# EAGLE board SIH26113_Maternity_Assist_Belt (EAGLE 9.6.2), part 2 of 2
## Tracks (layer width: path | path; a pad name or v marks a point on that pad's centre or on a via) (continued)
LED_STDBY_K  (via drill 0.3 pad 0.6)
  Top 0.2: 24.8,14.6 24.8,15 25,15.2 25,20 24.8,20.2 24.2,20.8 24,21 24,21.4 23.6,21.4 23.2,21.8 23,22 22.8,22.2 v22.4,22.6
  Top 0.25: U1.6 24.6,14.37
  Bottom 0.2: v22.4,22.6 22.2,22.8 22,23 21.8,23.2 21.2,23.8 21,24 20.8,24.2 v20.2,24.8
MOTOR_EN  (via drill 0.3 pad 0.6)
  Top 0.2: 69.6,59.6 69.6,59.8 69.8,60 70.2,60.4 70.4,60.6 70.6,60.8 70.8,61 71.2,61.4 71.2,64.4 71,64.6 70.8,64.8 | 23,45.6 23,47.4 22.8,47.6 22.6,47.8 22.4,48 v22.2,48.2 | v21.6,48.8 21.6,49 22,49.4 22.2,49.6 22.4,49.8 v22.4,55 | v22.4,55.8 22.6,56 23,56.4 23.2,56.6 23.4,56.8 23.6,57 24,57.4 24.2,57.6 24.4,57.8 24.6,58 v25,58.4 | v31,61.4 36.2,61.4 36.6,61.8 36.8,62 37.8,62 38,62.2 38.2,62.4 38.4,62.6 38.6,62.8 38.8,63 v41.2,63 | v56,62.6 67,62.6 67.2,62.8 67.4,63 67.6,63.2 67.8,63.4 68,63.6 68.2,63.8 68.4,64 68.6,64.2 68.8,64.4 69,64.6 69.2,64.8
  Top 0.25: U3.24 23.45,41.15
  Bottom 0.2: v22.2,48.2 22,48.4 21.8,48.6 v21.6,48.8 | v22.4,55 v22.4,55.8 | v25,58.4 25.2,58.6 25.4,58.8 25.6,59 26,59.4 26,60.4 29.8,60.4 30,60.6 30.2,60.8 30.4,61 30.8,61.4 v31,61.4 | v41.2,63 41.4,62.8 41.6,62.8 41.8,62.6 v56,62.6
MOTOR_G
  Top 0.2: 71.6,58.2 71.6,57.6 71.8,57.4 72,57.2 | 72,57.2 72,55.8 71.6,55.8 71.4,55.6 71.2,55.4 71,55.4 70.8,55.2 | 73.8,57.4 72.2,57.4 72,57.2
MOTOR_N
  Top 0.5: 83,62.8 83,64.8 84.4,66.2 | 75.2,60.6 81,60.6 81.2,60.8 81.4,61 81.8,61.4 82,61.6
MOTOR_P  (via drill 0.3 pad 0.6)
  Top 0.5: 80,64.8 80.4,64.8 80.8,65.2 81,65.4 81.2,65.6 81.4,65.8 81.8,66.2 82,66.4 82.2,66.6 82.4,66.8 82.8,67.2 83,67.4 83.2,67.6 83.4,67.8 83.8,68.2 84,68.4 85.6,68.4 85.8,68.2 86,68 86.2,67.8 86.4,67.6 86.4,67.4 | 75.6,62.4 75.6,62.2 77.8,62.2 78,62.4 78.2,62.6 78.6,62.6 78.8,62.8 78.8,63.2
  Bottom 0.5: v82,60.4 82,61.2 81.8,61.4 81.6,61.6 81.4,61.8 81.2,62 81,62.2 80.8,62.4 80.6,62.6 80.4,62.8 80.2,63 v80,63.2
PIEZO_AC  (via drill 0.3 pad 0.6)
  Top 0.2: 56.8,6.8 56.8,7.2 56.6,7.4 56.4,7.6 56.2,7.8 v56,8 | 57.2,17 v57.2,16.4 | 55,18.8 55.2,18.6 55.4,18.6 55.6,18.4 55.8,18.2 56,18.2
  Bottom 0.2: v56,8 55.8,8.2 55.8,10.4 v55.6,10.6 | v57.2,16.4 57.2,13.2 57,13 56.8,12.8 56.6,12.6 56.4,12.4 56.2,12.2 56,12 v55.6,12
PIEZO_ADC  (via drill 0.3 pad 0.6)
  Top 0.2: 58.8,14.4 v58.8,12.6 | 59.6,21.2 v60.2,21.2 | 54.6,21.8 v54.8,21.8 | 33.2,59.8 33.4,59.6 33.6,59.4 33.8,59.2 34,59 34.2,58.8 34.4,58.6 34.6,58.4 v34.8,58.2 | v48.2,61 53.6,61 53.8,60.8 v57.4,60.8 | v63.6,60.8 63.8,60.6 65.4,60.6 65.6,60.4 v65.6,55.8 | v65.6,25 65.2,25 65,25.2 64.8,25.4 63.6,25.4 63.4,25.2 63.2,25 63,24.8 62.8,24.6 62.6,24.4 62.4,24.2 62.2,24 62,23.8 61.8,23.6 61.6,23.4 61.4,23.2 61.2,23 61,22.8 60.8,22.6 60.6,22.4 59.6,22.4
  Top 0.25: U3.38 33.05,59.97
  Bottom 0.2: v58.8,12.6 58.8,12.2 58.6,12 v58.6,6.8 | v60.2,21.2 60.6,21.2 60.8,21 60.8,18.4 60.6,18.2 60.4,18 60,17.6 v60,15.6 | v54.8,21.8 v58.4,21.8 | v34.8,58.2 35,58 35.2,57.8 38.8,57.8 42.4,61.4 42.8,61.4 43.2,61.8 46.4,61.8 46.6,61.6 46.8,61.4 47,61.2 47.2,61 v48.2,61 | v57.4,60.8 v63.6,60.8 | v65.6,55.8 65.6,52.6 65.4,52.4 65,52 65,50.4 65.4,50 65.6,49.8 65.8,49.6 65.8,49 66,48.8 66.2,48.6 66.2,40.6 66,40.4 65.8,40.2 65.8,30 66.2,29.6 66.2,27.8 66,27.6 66,25.2 65.8,25 v65.6,25
PIEZO_IN  (via drill 0.3 pad 0.6)
  Top 0.2: 54.4,6.4 54.4,3.8 | 53.6,10.6 53.8,10.4 54,10.2 v54.2,10
  Bottom 0.2: v54.2,10 54.4,9.8 54.6,9.6 v54.6,7.6
SD_CS
  Top 0.25: U3.18 15.82,41.15
SD_MISO
  Top 0.25: U3.21 19.64,41.15
SD_MOSI  (via drill 0.3 pad 0.6)
  Top 0.2: 17.2,39.2 19.6,39.2 19.8,39 20,38.8 20.2,38.6 20.4,38.4 22.8,38.4 23,38.2 23.2,38 23.4,37.8 23.8,37.4 24,37.2 24.2,37 24.4,36.8 24.8,36.4 25,36.2 25.2,36 25.4,35.8 25.8,35.4 26,35.2 26.2,35 26.4,34.8 26.8,34.4 27,34.2 27.2,34 27.4,33.8 27.8,33.4 28,33.2 28.2,33 28.4,32.8 28.8,32.4 29,32.2 30.8,30.4 31,30.4 31.2,30.2 31.4,30 32,29.4 32.2,29.2 32.4,29 32.8,28.6 33,28.4 33.2,28.2 33.4,28 33.6,27.8 33.6,27.4 33.8,27.2 34,27 34,26.4 34.2,26.2 34.4,26 34.8,25.6 36.8,25.6 37,25.4 37.2,25.2 37.4,25 37.8,24.6 38,24.4 38.2,24.2 38.4,24 38.6,23.8 38.8,23.6 39,23.4 v39.2,23.2 | v42,22.4 42,24 42.2,24.2 42.4,24.4 42.6,24.6 42.8,24.8 v43,25 | v43.6,25.6 v45,25.6 | v52.4,23.2 55,23.2 55,25 55.2,25.2 55.4,25.4 55.6,25.6 55.8,25.8 56,26 56.2,26.2 56.4,26.4 56.6,26.6 56.8,26.8 57,27 57.2,27.2 57.4,27.4 57.6,27.6 57.8,27.8 58,28 58.2,28.2 58.4,28.4 58.6,28.6 58.8,28.8 59,29 59.2,29.2 59.4,29.4 59.6,29.6 59.8,29.8 60,30 60.2,30.2 60.4,30.4 60.6,30.6 v60.8,30.8 | v62.8,32 63,32.2 63.2,32.4 63.4,32.6 63.6,32.8 63.8,33 64,33.2 64.2,33.4 64.6,33.8 v64.6,48 | v64,59 63,59 62.8,59.2 62.4,59.6 62.2,59.6 61.6,60.2 61.4,60.4 61.2,60.6 60.6,61.2 60.4,61.4 60.2,61.6 59.8,62 53.4,62 51,64.4 50.8,64.6 50.6,64.8 50.4,64.8 50.2,65 49.6,65 49.4,65.2 v49.2,65.4
  Top 0.25: U3.19 17.09,39.45
  Bottom 0.2: v39.2,23.2 39.4,23 39.6,22.8 39.8,22.6 40,22.4 40.2,22.2 40.4,22 40.6,21.8 40.8,21.6 42,21.6 v42,22.4 | v43,25 43.2,25.2 43.4,25.4 v43.6,25.6 | v45,25.6 50,25.6 50.4,25.2 50.6,25 50.8,24.8 51,24.6 51.4,24.2 51.6,24 51.8,23.8 52,23.6 v52.4,23.2 | v60.8,30.8 61,31 61.2,31.2 61.4,31.4 61.6,31.6 61.8,31.8 62,32 v62.8,32 | v64.6,48 64.6,49.6 64.4,49.8 64.4,58.6 64.2,58.8 v64,59 | v49.2,65.4 49,65.6 48.8,65.8 48.6,66 48.4,66.2 48,66.6
SD_SCK  (via drill 0.3 pad 0.6)
  Top 0.2: v17.8,46.8 18.6,46.8 18.8,47 20.4,47 20.8,47.4 21,47.6 21.2,47.8 21.4,48 21.8,48.4 22,48.6 22.2,48.8 22.4,49 22.8,49.4 23,49.6 23.2,49.8 23.4,50 23.8,50.4 24,50.6 24.2,50.8 24.4,51 24.8,51.4 v25,51.6
  Top 0.25: U3.20 18.36,42.85
  Bottom 0.2: v18,45.6 18,46.4 17.8,46.6 v17.8,46.8 | v25,51.6 25.2,51.8 25.4,52 25.8,52.4 26,52.6 27.4,52.6 27.6,52.8 27.8,53 28,53.2 28.2,53.4 28.4,53.6 28.6,53.8 28.8,54 29,54.2 29.2,54.4 29.4,54.6 29.6,54.8 29.8,55 30,55.2 30.2,55.4 30.4,55.6 30.6,55.8 30.8,56 31,56.2 31.2,56.4 31.4,56.6 31.6,56.8 31.8,57 32,57.2 32.6,57.8 32.8,58 33,58.2 33.6,58.8 33.8,59 34,59.2 34.6,59.8 34.8,60 35,60.2 35.2,60.2 35.4,60.4 37,60.4 37.2,60.6 37.4,60.8 37.6,61 37.8,61.2 38,61.4 38.2,61.6 38.8,62.2 39,62.4 39.2,62.6 39.8,63.2 40,63.4 40.2,63.6 40.8,64.2 41,64.4 41.2,64.6 41.4,64.8 41.6,64.8 41.8,65 42.4,65 42.6,65.2 42.8,65.4 43,65.6 43.2,65.8 43.4,66 43.6,66.2 43.8,66.4 44,66.6
SOS_BTN
  Top 0.2: 49.6,57.4 49.6,58.2 49.8,58.4 | 52.8,55.2 49.8,55.2 49.8,55.8 49.6,56 | 58,61.6 52.8,61.6 50.6,63.8
SOS_GPIO  (via drill 0.3 pad 0.6)
  Top 0.2: 51.6,57.4 51.6,57.6 v53.4,59.4 | 29.8,53.8 v33,53.8
  Top 0.25: U3.33 29.65,53.62
  Bottom 0.2: v53.4,59.4 56.8,62.8 57,62.8 57.2,63 57.2,63.2 57.4,63.4 57.4,63.6 57.6,63.8 57.8,64 v58,64.2 | v33,53.8 48.2,53.8 48.4,54 48.6,54.2 49.2,54.8 49.4,55 49.6,55.2 50.2,55.8 v50.4,56
STRETCH_ADC  (via drill 0.3 pad 0.6)
  Top 0.2: 58.8,10.2 59.6,10.2 59.8,10.4 60,10.6 60.2,10.8 | 56.8,13 56.8,10.4 57,10.4 57.2,10.2 | v31.6,31.2 31.8,31 32,30.8 32.2,30.6 32.4,30.4 32.6,30.2 32.8,30 33,29.8 33.2,29.6 33.4,29.4 33.6,29.2 33.8,29 34,28.8 34.2,28.6 34.4,28.4 34.6,28.2 34.8,28 37,28 37.2,27.8 37.4,27.6 37.8,27.2 38,27 38.4,26.6 38.6,26.4 38.8,26.2 39,26 39.4,25.6 39.6,25.4 39.8,25.2 40,25 v40.2,24.8 | v43.6,21.4 43.8,21.2 44,21 v44.2,20.8
  Top 0.25: U3.12 4.95,48.54
  Bottom 0.2: v11,48 14.8,48 15,47.8 15.2,47.6 15.4,47.4 15.6,47.2 15.8,47 16,46.8 16.2,46.6 16.4,46.4 16.8,46 17,45.8 17.2,45.6 17.4,45.4 17.8,45 18,44.8 18.2,44.6 18.4,44.4 18.8,44 19,43.8 19.2,43.6 19.4,43.4 19.8,43 20,42.8 20.2,42.6 20.4,42.4 20.8,42 21,41.8 21.2,41.6 21.4,41.4 21.8,41 22,40.8 22.2,40.6 22.4,40.4 22.8,40 23,39.8 23.2,39.6 23.4,39.4 23.8,39 24,38.8 24.2,38.6 24.4,38.4 24.8,38 25,37.8 25.2,37.6 25.4,37.4 25.6,37.2 25.8,37 26,36.8 26.2,36.6 26.4,36.4 26.6,36.2 26.8,36 27,35.8 27.2,35.6 27.4,35.4 27.6,35.2 27.8,35 28,34.8 28.2,34.6 28.4,34.4 28.6,34.2 28.8,34 29,33.8 29.2,33.6 29.4,33.4 29.6,33.2 29.8,33 30,32.8 30.2,32.6 30.4,32.4 30.6,32.2 30.8,32 31,31.8 31.2,31.6 v31.6,31.2 | v40.2,24.8 40.4,24.6 40.6,24.4 40.8,24.2 41,24 41.4,23.6 41.6,23.4 41.8,23.2 42,23 42.4,22.6 42.6,22.4 42.8,22.2 43,22 43.4,21.6 v43.6,21.4 | v44.2,20.8 46.4,20.8 46.6,20.6 46.8,20.4 47,20.2 47.2,20 47.4,19.8 47.6,19.6 47.8,19.4 48,19.2 48.2,19 48.4,18.8 48.6,18.6 48.8,18.4 49,18.2 49.4,17.8 49.6,17.6 49.8,17.4 50,17.2 50.4,16.8 50.6,16.6 50.8,16.4 51,16.2 51.4,15.8 51.6,15.6 51.8,15.4 52,15.2 52.2,15 52.4,14.8 55.6,14.8 55.8,14.6 56,14.4 v56.2,14.2
TMP_ALERT  (via drill 0.3 pad 0.6)
  Top 0.2: U4.3 51,38.85 49.6,38.35 | 54.8,48 54.6,48.2 54,48.2 54,49 53.8,49.2 53.2,49.8 53,50 52.8,50.2 52.2,50.8
  Bottom 0.2: v51.8,39 51.8,43.8 v54.8,46.8
UART_RX  (via drill 0.3 pad 0.6)
  Top 0.2: 29.8,57.2 32,57.2 32.4,56.8 v33,56.8 | v59,56.8 59.4,56.8 59.6,56.6 59.6,50 59.8,49.8 60,49.6 v60,48.8 | v61.2,39.2 61.2,35.8 61.4,35.6 61.6,35.4 v61.6,33.2 | v57.6,30.8 57.4,30.6 57,30.2 v56.8,30.2 | v44.4,27.2 43,27.2 42.8,27.4 42.6,27.6 v42.4,27.8 | v35.4,30.8 35.2,30.8 35,31 34.8,31.2 v34.6,31.2 | v28.6,24.8 28.6,24.6 v27,24.6 | v25,24 18,24 17.8,24.2 17.4,24.6 15.2,24.6 15,24.8 14.8,25 v13,25 | v10.8,25 8.8,25 8.6,25.2 8.2,25.6 8,25.8 7.8,26 7.6,26.2 7,26.8 6.8,27 6.6,27.2 6,27.8 5.8,28 5.6,28.2 5,28.8 4.8,29 4.6,29.2 4,29.8 3.8,30 3.6,30.2 3.4,30.4 3,30.8
  Top 0.25: U3.36 29.65,57.43
  Bottom 0.2: v33,56.8 33.4,56.8 33.6,56.6 33.8,56.4 34,56.2 34.6,55.6 34.8,55.4 35,55.2 35.2,55.2 35.4,55 48.2,55 48.4,55.2 48.6,55.4 48.8,55.6 49,55.8 49.2,56 49.4,56.2 49.6,56.4 49.8,56.6 57.4,56.6 57.6,56.8 v59,56.8 | v60,48.8 60,40.4 v61.2,39.2 | v61.6,33.2 60.8,33.2 60.4,32.8 59.6,32.8 59.4,32.6 59.2,32.4 59,32.2 58.8,32 58.6,31.8 58.4,31.6 58,31.2 57.8,31 v57.6,30.8 | v56.8,30.2 49.8,30.2 49.6,30 49.4,29.8 49.2,29.6 48.2,29.6 48,29.4 47.8,29.2 47.6,29 47.4,28.8 47,28.4 46.8,28.2 46.6,28 46.4,27.8 46,27.4 45.8,27.2 v44.4,27.2 | v42.4,27.8 42.2,28 42,28.2 41.8,28.4 41.6,28.6 41.4,28.8 41.2,29 41,29.2 40.8,29.4 40.6,29.6 39.8,29.6 39.6,29.8 39.6,30.4 37.2,30.4 37,30.6 36.8,30.8 v35.4,30.8 | v34.6,31.2 34.4,31 34.2,30.8 34,30.6 33.8,30.4 33.6,30.2 33.4,30 33.2,29.8 33,29.6 32.8,29.4 32.6,29.2 32.4,29 32.2,28.8 32,28.6 31.6,28.2 31.4,28 31.2,27.8 31,27.6 30.6,27.2 30.4,27 30.2,26.8 30,26.6 29.6,26.2 29.4,26 29.2,25.8 29,25.6 28.6,25.2 v28.6,24.8 | v27,24.6 25.6,24.6 v25,24 | v13,25 v10.8,25
UART_TX  (via drill 0.3 pad 0.6)
  Top 0.2: 27,58.8 v11.4,58.8
  Top 0.25: U3.37 31.35,58.7
  Bottom 0.2: v11.4,58.8 8.8,58.8 8.8,42.4 8.6,42.2 8.4,42 8.4,35.4 8.2,35.2 8,35 7.8,34.8 7.4,34.4 7.2,34.2 7,34 6.8,33.8 6.4,33.4 6.2,33.2 6,33 5.8,32.8 5.4,32.4 5.2,32.2 5,32 4.8,31.8 4.2,31.2 4,31 3.8,30.8 3.6,30.6 3.4,30.4 3.2,30.2 3,30 2.8,29.8 2.6,29.6
USB_DM  (via drill 0.3 pad 0.6)
  Top 0.2: 9.6,46.8 9.2,46.8 v9.2,41.4
  Bottom 0.2: v9.2,41.4 9.2,5 9.4,4.8 9.6,4.6 10,4.2 10.2,4 10.4,3.8
USB_DP  (via drill 0.3 pad 0.6)
  Top 0.2: 10.4,40.6 v10.4,40.2
  Top 0.25: U3.14 10.25,40.7
  Bottom 0.2: v10.4,40.2 10.4,23.2 10.6,23 10.8,22.8 10.8,21 11,20.8 11.2,20.6 11.4,20.4 11.6,20.2 11.6,5 11.8,4.8 12,4.6 12.2,4.4 12.4,4.2 12.6,4 12.8,3.8
VBAT  (via drill 0.3 pad 0.6)
  Top 0.25: U1.5 24.6,13.1
  Top 0.5: 22,12.8 22,5.4 21.6,5 21.4,4.8 21.2,4.6 21,4.4 20.6,4 20.4,3.8 | 15.2,15.4 v16,15.4 | 10,17.6 10,17.2 10.2,17 13.2,17 13.4,16.8 13.6,16.8 13.8,16.6 | 8.6,21 8.6,20 8.8,19.8 9,19.6 9.2,19.4 9.4,19.2 9.6,19 9.8,18.8 | 14.4,27.4 14.2,27.2 14,27 13.6,26.6 13.4,26.4 13.2,26.2 13,26 12.6,25.6 12.4,25.4 12.2,25.2 12,25 11.6,24.6 11.4,24.4 11.2,24.2 11,24 10.6,23.6 10.4,23.4 10.2,23.2 10,23 9.4,23 9.2,22.8 9.2,22.4 9,22.2 8.6,22.2 | 16.8,31.2 16.6,31 16.4,30.8 v16.2,30.8 | 24.4,27.6 21.8,27.6 21.4,28 21.2,28.2 21,28.4 20.4,29 20.2,29.2 20,29.4 19.4,30 19.2,30.2 19,30.4 18.2,31.2 | 2.6,49.4 2.6,47 2.8,46.8 3,46.6 3.2,46.4 3.4,46.2 3.6,46 3.8,45.8 4,45.6 4.2,45.4 4.6,45 4.8,44.8 5,44.6 5.2,44.4 5.6,44 5.8,43.8 6,43.6 6.2,43.4 6.6,43 6.8,42.8 7,42.6 7.2,42.4 7.6,42 7.8,41.8 8,41.6 8.2,41.4 8.6,41 8.8,40.8 9,40.6 9.2,40.4 9.4,40.2 9.6,40 9.8,39.8 10,39.6 10.2,39.4 10.4,39.2 10.6,39 10.8,38.8 11,38.6 11.2,38.4 11.4,38.2 11.6,38 11.8,37.8 12,37.6 12.2,37.4 12.4,37.2 12.6,37 12.8,36.8 13,36.6 13.2,36.4 13.4,36.2 13.6,36 13.8,35.8 14,35.6 14.2,35.4 14.4,35.2 14.6,35 14.8,34.8 15,34.6 15.2,34.4 15.4,34.2 15.6,34 15.8,33.8 16.2,33.4 16.4,33.2 16.6,33 16.8,32.8 | 77,63.2 v76.2,63.2
  Bottom 0.5: v16,15.4 17.2,15.4 17.4,15.2 17.6,15 18,14.6 18.2,14.4 18.4,14.2 18.6,14 19,13.6 19.2,13.4 v22,13.4 | v16.2,30.8 15.8,30.8 15.6,30.6 v15.6,28.6 | v76.2,63.2 67.2,63.2 67,63 66.8,62.8 66.6,62.6 66.4,62.4 66,62 65.8,61.8 65.6,61.6 65.4,61.4 65,61 64.8,60.8 64.6,60.6 64.4,60.4 41.6,37.6 41.4,37.4 41.2,37.2 40.6,36.6 40.4,36.4 40.2,36.2 39.6,35.6 37,35.6 36.8,35.4 36.6,35.2 36,34.6 35.8,34.4 35.6,34.2 35,33.6 34.8,33.4 34.6,33.2 34,32.6 33.8,32.4 33.6,32.2 33.4,32 33.2,31.8 33,31.6 32.8,31.4 32.6,31.2 32.4,31 32.2,30.8 32,30.6 31.6,30.2 31.4,30 31.2,29.8 31,29.6 30.6,29.2 30.4,29 30.2,28.8 30,28.6 29.6,28.2 28.6,28.2 28.4,28 28.2,27.8 25.8,27.8 v25.6,27.6
VBAT_SENSE
  Top 0.2: 25.6,23.6 26,24 26,24.2 26.2,24.4 26.8,25 | 25.6,28.4 26.4,28.4 26.4,26.4 26.6,26.2 26.8,26.2 | 14.8,42.6 14.8,40.8 15,40.6 15.2,40.4 15.4,40.2 15.6,40 15.8,39.8 16,39.6 16.2,39.4 16.4,39.2 16.6,39 16.8,38.8 17,38.6 17.2,38.4 17.4,38.2 17.6,38 17.8,37.8 18.2,37.4 18.4,37.2 18.6,37 18.8,36.8 19,36.6 19.2,36.4 19.4,36.2 19.6,36 19.8,35.8 20,35.6 20.2,35.4 20.4,35.2 20.6,35 20.8,34.8 21,34.6 21.2,34.4 21.4,34.2 21.6,34.2 21.6,33.8 22,33.4 22.2,33.2 22.2,31.8 22.8,31.2 23,31 23.2,30.8 23.8,30.2 24,30 24.2,29.8 24.4,29.6
  Top 0.25: U3.17 14.55,42.85
VBUS  (via drill 0.3 pad 0.6)
  Top 0.25: U1.4 15.4,13.1 | U1.8 24.6,16.91
  Top 0.5: 12.4,11.4 12.4,7.6 12.2,7.4 12,7.2 11.8,7 11.6,6.8 11.4,6.6 11.2,6.4 11,6.2 10.8,6 10.6,5.8 10.4,5.6 10.2,5.4 10,5.2 9.8,5 9.6,4.8 9.4,4.6 9.2,4.4 9,4.2 8.8,4 8.6,3.8 | 15.2,12.8 13.8,12.8 13.6,12.6 | 22,16.6 21.6,16.6 21.4,16.4 21.2,16.2 21,16 20.6,15.6 20.4,15.4 20.2,15.2 20,15 v19.6,14.6 19.4,14.4 19.2,14.2 19,14 18.6,13.6 18.4,13.4 18,13.4 | 14,22.8 14,21.2 | 14,31.6 v14,31
  Bottom 0.5: v15.2,19.8 15.4,19.8 15.4,19 15.6,18.8 16,18.4 16.2,18.2 16.2,18 16.4,17.8 16.8,17.4 17,17.2 17.2,17 17.4,16.8 17.8,16.4 18,16.2 18.2,16 18.4,15.8 18.6,15.6 18.8,15.4 19,15.2 19.2,15 v19.6,14.6 | v14,31 v14,24.2

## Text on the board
tPlace: SIH26113 MATERNITY ASSIST BELT rev A | NOT A MEDICAL DEVICE - PROTOTYPE ONLY
bPlace: 4-LAYER FR-4 1.6mm 1oz Cu L2=GND L15=3V3
Document: Z2 ESP32-S3 CORE | Z7 USER INPUT / STORAGE | Z6 FET-DRIVEN ALERTS | ANTENNA KEEPOUT - NO COPPER / NO PLANE / NO PARTS | Z4 I2C SENSORS | Z3 ECG ANALOG FRONT END | Z1 POWER ENTRY / CHARGING / 3V3 | Z5 MECHANICAL SENSING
